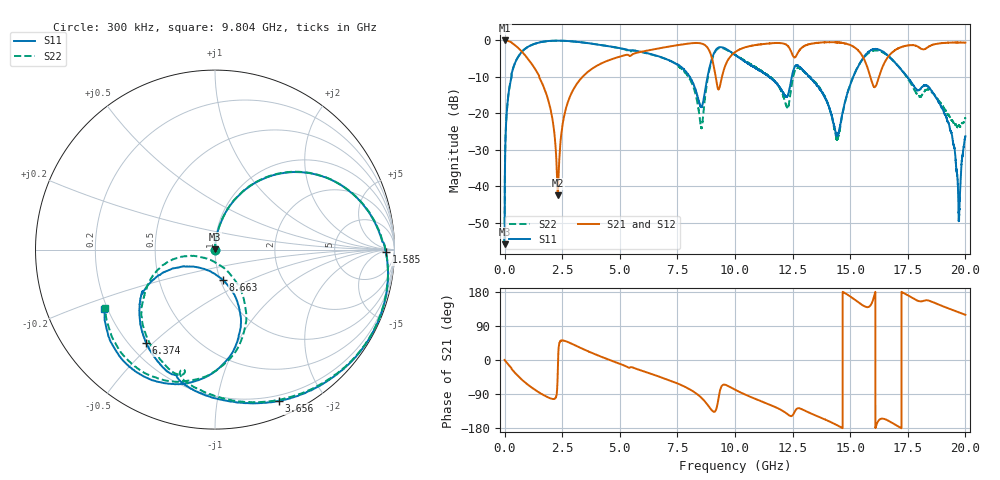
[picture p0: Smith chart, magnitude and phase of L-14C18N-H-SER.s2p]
!{L-14C18N}
!Johanson Technology Inc.
!www.johansontechnology.com
!Test Board Conditions:
!Substrate Type  RO4350B
!Substrate Thickness  20 mil
!Substrate Dk  3.66
!TL Type: GCPW
!TL Trace Width  36 mil
!TL Gap  12 mil
!Electrode orientation  Horizontal
!DUT TOPOLOGY	SERIES
!Mounting Pad LxW  26x36 mil
! Created Sun Jun 20 13:02:21 2021
# hz S ma R 50
! 2 Port Network Data from SP1.SP block
! freq  magS11  angS11  magS21  angS21  magS12  angS12  magS22  angS22
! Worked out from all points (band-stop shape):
!   20001 points, 300 kHz to 20 GHz, reference 50 ohm
!   highest |S21| = 0.00 dB at 14.3 MHz (marker M1); lowest = -42.5 dB at 2.311 GHz (marker M2)
!   |S21| within 3 dB of the highest: 6.015 GHz to 8.899 GHz (2.884 GHz wide, 38.7 % of centre); 16.88 GHz to end of sweep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
!   lowest |S11| = -55.9 dB at 1.3 MHz (marker M3), VSWR 1.00, Z = 49.9 + j0.0688 ohm
!   |S11| at or under -10 dB: 11.49 GHz to 12.47 GHz (972.3 MHz wide, 8.12 % of centre); 13.24 GHz to 15.13 GHz (1.887 GHz wide, 13.3 % of centre); 17.48 GHz to end of sweep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
!   |S22| runs from -56.4 to -0.1 dB; largest |S21 - S12| = 0.016
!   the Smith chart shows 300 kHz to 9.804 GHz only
!   S11 on the Smith chart (normalised r, x): 300 kHz: 1.00, -0.00; 1.585 GHz: 37, -11; 3.656 GHz: 0.14, -1.50; 6.374 GHz: 0.27, -0.48; 8.663 GHz: 1.03, -0.36; 9.804 GHz: 0.19, -0.24
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300000  0.001719 -118.7  0.9993 0.1  0.9986 0.1  0.002001 -128.0
1300000  0.001605 154.6  0.9987 -0.0  0.9986 -0.1  0.001513 144.8
1.43e7  0.01721 89.2  0.9997 -1.1  0.9996 -1.1  0.01741 89.4
1.293e8  0.1426 78.7  0.9857 -9.6  0.9858 -9.6  0.1434 78.9
3.753e8  0.4201 60.0  0.8976 -28.7  0.8973 -28.7  0.4224 60.1
1.5853e9  0.9519 -0.8  0.2763 -88.9  0.2773 -88.8  0.9515 -0.5
2.3113e9  0.9929 -26.0  0.007508 -20.0  0.007524 -20.1  0.9921 -25.3
3.3343e9  0.9436 -58.0  0.305 31.0  0.3061 31.0  0.9416 -56.6
3.6563e9  0.9156 -67.0  0.3797 22.2  0.3803 22.2  0.9142 -65.5
6.3743e9  0.6458 -126.3  0.7453 -36.9  0.7475 -36.8  0.6398 -123.9
6.6673e9  0.6075 -132.1  0.7752 -43.1  0.777 -42.9  0.6039 -130.3
8.6633e9  0.173 -75.7  0.8767 -107.2  0.8765 -107.2  0.1297 -61.1
9.2163e9  0.7733 -104.4  0.247 -123.3  0.2498 -123.3  0.7514 -102.9
9.8043e9  0.7006 -151.6  0.6052 -71.7  0.6097 -71.7  0.6915 -151.9
1.00003e10  0.6347 -160.3  0.6911 -78.3  0.693 -78.2  0.6365 -160.8
1.33343e10  0.2919 133.7  0.9036 -142.2  0.9006 -142.2  0.2968 137.9
1.44463e10  0.05011 178.4  0.9391 -172.6  0.9401 -172.6  0.04344 -172.2
1.55303e10  0.5564 -156.5  0.6084 145.0  0.613 144.2  0.5472 -142.9
1.66673e10  0.6045 122.4  0.6101 -160.6  0.608 -159.3  0.6096 132.0
1.89593e10  0.1213 60.8  0.9176 143.4  0.9196 143.4  0.1324 81.3
1.97053e10  0.004344 111.4  0.9364 125.8  0.9357 126.1  0.06808 116.3
2e10  0.04865 -151.0  0.9337 119.2  0.9278 119.1  0.08654 147.7
